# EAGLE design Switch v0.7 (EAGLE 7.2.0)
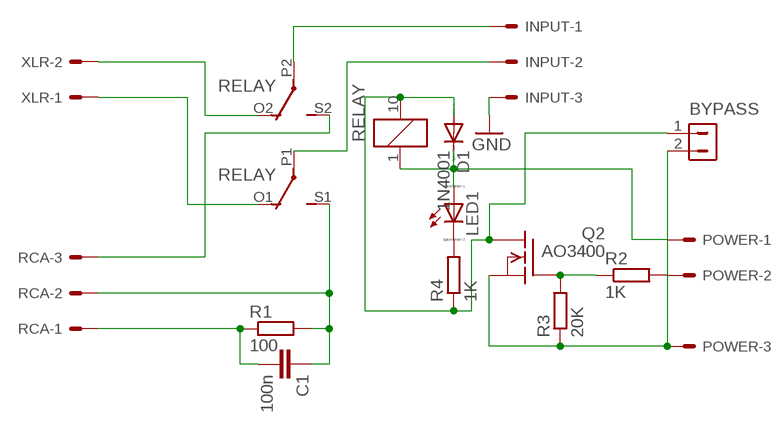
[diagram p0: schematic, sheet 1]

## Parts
BYPASS  CON-2  [CON-2]
C1  100n  C-EU050-025X075  [C050-025X075]
D1  1N4001  DIODE-DO214BA  [DO214BA]
INPUT  22-27-2031-03  [6410-03]
LED1  LED_E  [LED_1206]
POWER  22-27-2031-03  [6410-03]
Q2  AO3400  [TRANSISTOR-PNP_SOT23-BEC]
R1  100  R-EU_0207/10  [0207/10]
R2  1K  RCL_R-EU_R1206  [RCL_R1206]
R3  20K  RCL_R-EU_R1206  [RCL_R1206]
R4  1K  RCL_R-EU_R1206  [RCL_R1206]
RCA  22-27-2031-03  [6410-03]
RELAY  G6H2-100  [G6H2-100]
XLR  22-27-2021-02  [6410-02]

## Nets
GND: INPUT.3
N$1: RELAY.O2(3:O) XLR.2
N$2: RELAY.O1(2:O) XLR.1
N$3: RCA.3 RELAY.S2(3:S)
N$4: C1.1 R1.2 RCA.2 RELAY.S1(2:S)
N$5: C1.2 R1.1 RCA.1
N$6: INPUT.1 RELAY.P2(3:P)
N$7: INPUT.2 RELAY.P1(2:P)
N$8: POWER.2 R2.2
N$9: D1.C LED1.A POWER.1 RELAY.1
N$10: LED1.C R4.2
N$11: BYPASS.2 POWER.3 Q2.E(S) R3.1
N$12: Q2.B(G) R2.1 R3.2
N$13: BYPASS.1 D1.A Q2.C(D) R4.1 RELAY.10

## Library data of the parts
BYPASS = Dimdim:CON-2
C1 = rcl:C-EU: CAPACITOR, European symbol
D1 = diode:DIODE-: DIODE
INPUT POWER RCA = con-molex:22-?-03: CONNECTOR wire to board 2.54 mm (.1 inch) pitch header; OC_FARNELL: unknown; OC_NEWARK: unknown
LED1 = eagle-ltspice:LED_E: LED; SPICEMODEL: NONE; SPICEPREFIX: D; SPICETYPE: diode
Q2 = Dimdim:AO3400
R1 = rcl:R-EU_: RESISTOR, European symbol
R2-R4 = Univ USBtoI2S indicator v0.8b:RCL_R-EU_: RESISTOR, European symbol
RELAY = relay:G6H2-100: RELAY 2 x switch, 0.5 A/125 V AC, 1 A/30 V DC, Omron; OC_FARNELL: unknown; OC_NEWARK: unknown
XLR = con-molex:22-?-02: CONNECTOR; OC_FARNELL: unknown; OC_NEWARK: unknown

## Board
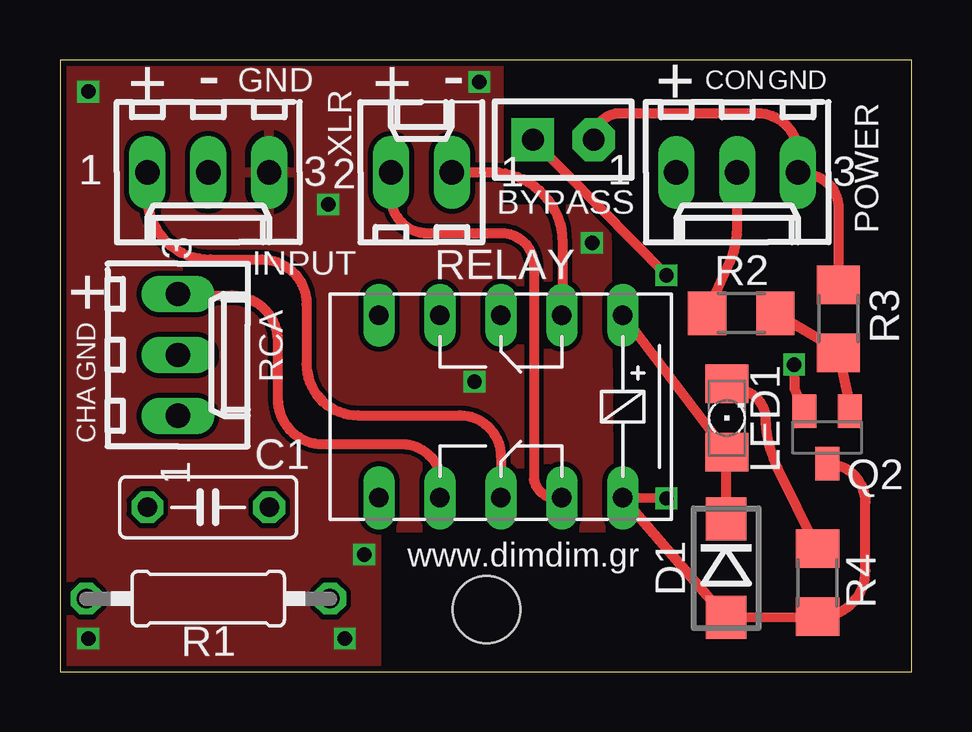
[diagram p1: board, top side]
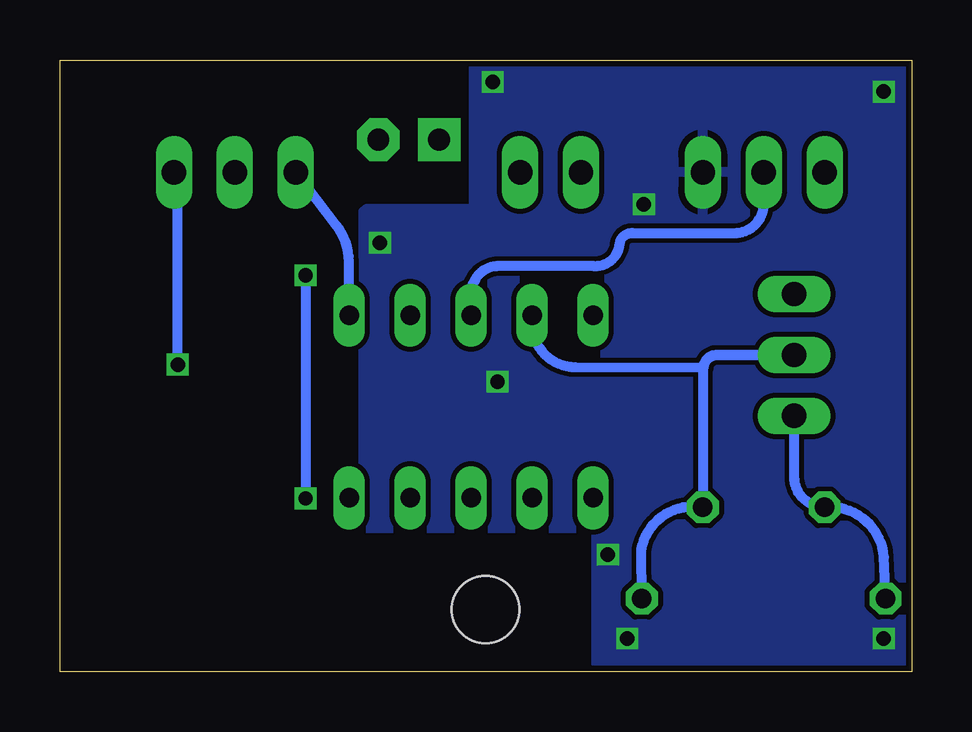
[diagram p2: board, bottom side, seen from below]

Size 35.52 x 25.5 mm. Coordinates in mm from the lower left corner, seen from the top.
Outline: 0,0 35.52,0 35.52,25.5 0,25.5 0,0
Copper layers (1*16): Top 0.035mm / dielectric 1.5mm / Bottom 0.035mm
Design rules "dirt_cheap_dirty_boards.v1 *": minimum track width 5mil, minimum drill 12mil, track to track 8mil, track to pad 8mil, pad to pad 8mil, via to via 5mil, smd to smd 0mil, copper to edge 10mil, drill to drill 10mil, minimum pad ring 10mil, minimum via ring 6mil, stop-mask expansion 2mil, vias tented up to drill 25mil, thermal gap 10mil
Holes 2.8 mm at 17.78,2.58

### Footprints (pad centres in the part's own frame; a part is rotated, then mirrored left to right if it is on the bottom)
CON-2 = drill 0.914 pad 1.778 square: 1 -1.27,0 | drill 0.914 pad 1.778 octagon: 2 1.27,0
C050-025X075 = drill 0.813 octagon: 1 -2.54,0; 2 2.54,0
DO214BA = smd 1.8 x 1.7: A 2.05,0; C -2.05,0
6410-03 = drill 1.016 long: 1 2.54,0; 2 0,0; 3 -2.54,0
LED_1206 = smd 1.6 x 1.803: A -1.422,0; C 1.422,0
TRANSISTOR-PNP_SOT23-BEC = smd 1 x 1.4: B -0.95,-1.1; C 0,1.1; E 0.95,-1.1
0207/10 = drill 0.813 octagon: 1 -5.08,0; 2 5.08,0
RCL_R1206 = smd 1.6 x 1.803: 1 -1.422,0; 2 1.422,0
G6H2-100 = drill 0.813 long: 1 -5.08,-3.81; 5 5.08,-3.81; 6 5.08,3.81; 10 -5.08,3.81; O1 -2.54,-3.81; O2 -2.54,3.81; P1 0,-3.81; P2 0,3.81; S1 2.54,-3.81; S2 2.54,3.81
6410-02 = drill 1.016 long: 1 1.27,0; 2 -1.27,0

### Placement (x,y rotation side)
BYPASS  20.98,22.18 0 top
C1  6.18,6.85 180 top
D1  27.77,4.31 270 top
INPUT  6.18,20.82 180 top
LED1  27.8,10.57 90 top
POWER  28.23,20.82 180 top
Q2  31.98,9.76 180 top
R1  6.18,3.04 0 top
R2  28.4,14.94 180 top
R3  32.45,14.71 270 top
R4  31.58,3.71 90 top
RCA  4.91,13.2 270 top
RELAY  18.38,11.05 180 top
XLR  15.07,20.82 0 top

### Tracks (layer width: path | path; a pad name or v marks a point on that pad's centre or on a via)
GND  (via drill 0.6)
  other vias: 11.88,1.38 1.18,1.38 12.68,4.88 17.28,12.08 17.48,24.58 1.18,24.18 11.18,19.48 22.18,17.88
  pour Top: 0.18,25.38 18.28,25.28 18.28,19.28 22.78,19.28 22.88,5.98 13.18,5.98 13.18,0.28 0.18,0.28
  pour Bottom: 0.18,25.38 18.28,25.38 18.28,19.28 22.78,19.28 22.78,19.18 22.88,19.18 22.88,5.98 13.18,5.98 13.18,0.38 0.18,0.18
N$1
  Top 0.406: XLR.2 13.8,19.78 arc90 15.3,18.28 18.41,18.28 arc-90 19.75,16.94 19.75,8.01 arc90 RELAY.O2
N$2
  Top 0.406: XLR.1 18.02,20.82 arc-90 20.95,17.89 20.95,17.09 RELAY.O1
N$3
  Top 0.406: RCA.3 4.91,15.68 7.16,15.68 arc-90 9.08,13.76 9.08,11.36 arc90 10.96,9.48 14.27,9.48 arc-90 15.88,7.87 15.88,7.24 RELAY.S2
N$4
  Bottom 0.406: R1.2 11.29,5.08 arc90 C1.1 8.72,12.58 arc90 8.1,13.2 RCA.2 8.16,13.2 arc-90 8.68,12.68 14.04,12.69 arc90 15.84,14.5 RELAY.S1
N$5
  Bottom 0.406: R1.1 1.17,4.78 arc-90 C1.2 arc90 4.91,8.12 RCA.1
N$6
  Top 0.406: INPUT.1 3.64,19.81 arc90 6.27,17.18 8.42,17.18 arc-90 10.28,15.32 10.28,12.82 arc90 12.42,10.68 16.68,10.68 arc-90 18.38,8.98 RELAY.P2
N$7
  Bottom 0.406: RELAY.P1 18.38,15.75 arc90 17.22,16.91 13.3,16.91 arc-90 12.19,17.82 arc90 11.63,18.28 7.4,18.28 arc-90 6.18,19.5 INPUT.2
N$8
  Top 0.406: R2.2 27.93,17.07 arc24 28.23,18.47 POWER.2
N$9
  Top 0.406: D1.C LED1.A RELAY.1
  Bottom 0.406: RELAY.1 23.48,17.1 arc-34 23.91,18.49 23.98,18.58 POWER.1
N$10
  Top 0.406: R4.2 29.91,8.5 arc-23 29.43,10.36 29.42,10.59 arc66 28.64,11.67 LED1.C
N$11  (via drill 0.6)
  Top 0.406: R3.1 32.45,19.44 arc90 30.97,20.72 POWER.3 30.77,21.58 arc90 29.07,23.28 23.35,23.28 arc90 BYPASS.2 | Q2.E 30.63,11.78 v30.61,12.8
  Bottom 0.406: v30.61,12.8 30.61,20.47 arc21 30.64,20.61 POWER.3
N$12
  Top 0.406: R2.1 32.38,13.44 R3.2 32.93,11.09 Q2.B
N$13  (via drill 0.6)
  Top 0.406: Q2.C arc-90 33.58,7.06 33.58,4.2 arc-90 31.66,2.29 R4.1 D1.A RELAY.10 v25.28,7.22 | BYPASS.1 v25.28,16.53
  Bottom 0.406: v25.28,16.53 v25.28,7.22

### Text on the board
tNames: + | - | + | - | + | GND | CON | GND | + | GND | CHA | www.dimdim.gr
